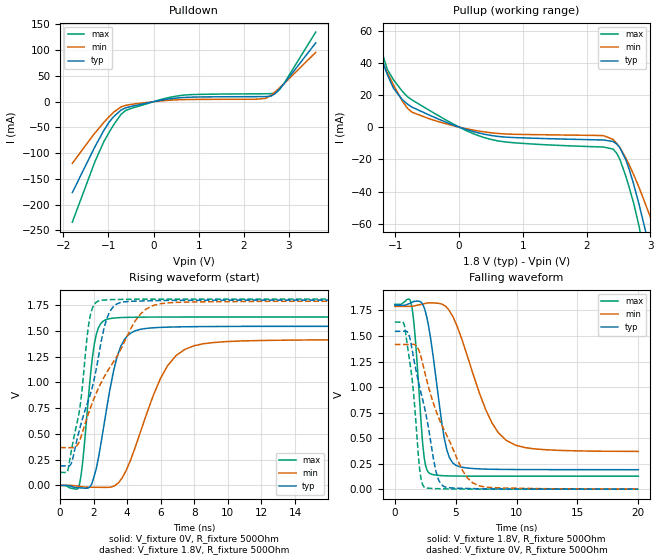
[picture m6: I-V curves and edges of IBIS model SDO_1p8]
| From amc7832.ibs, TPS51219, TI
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|   Model
[Model]   SDO_1p8
Model_type   Output
Polarity   Non-Inverting
Vmeas = 0.9
Vref = 0
Cref = 1pF
Rref = 100000
|   typ   min   max
C_comp   1pF   1pF   1pF
[Voltage Range]   1.8   1.79   1.81
[Temperature Range]   27   125   -40
[Pullup Reference]   1.8   1.79   1.81
[Pulldown Reference]   -0   -0   -0
[Power Clamp Reference]   1.8   1.79   1.81
[GND Clamp Reference]   -0   -0   -0
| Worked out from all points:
|   slope of the pulldown table from 0 to 0.27 V, typ, clamps not added: 62.1 ohm
|   slope of the pullup table from 0 to 0.27 V, typ, clamps not added: 83.4 ohm
|   falling waveform, V_fixture 1.8V, R_fixture 500Ohm: 20-80 % time 1.1ns typ, 2.57ns min, 595ps max; typ from 1.8 V to 0.19 V
|   rising waveform, V_fixture 0V, R_fixture 500Ohm: 20-80 % time 1.05ns typ, 2.02ns min, 575ps max; typ from 0 V to 1.54 V
|   rising waveform, V_fixture 1.8V, R_fixture 500Ohm: 20-80 % time 1.45ns typ, 2.57ns min, 813ps max; typ from 0.191 V to 1.8 V
|   falling waveform, V_fixture 0V, R_fixture 500Ohm: 20-80 % time 1.54ns typ, 2.68ns min, 785ps max; typ from 1.54 V to 0 V
[Pulldown]
|   Voltage   I(typ)   I(min)   I(max)
-1.8V     -176.6mA   -119.8mA   -234.2mA
-1.319V   -91.03mA   -63.11mA   -121.2mA
-1.103V   -56.2mA    -40.42mA   -78.11mA
-882mV    -29.02mA   -20.34mA   -44.72mA
-725.4mV  -16.76mA   -10.41mA   -25.13mA
-617.4mV  -11.91mA   -7.125mA   -16.98mA
608.4mV   7.777mA    3.867mA    12.1mA
2.266V    9.812mA    4.73mA     15.25mA
2.482V    9.901mA    6.398mA    15.37mA
2.704V    16.5mA     19.76mA    17.88mA
2.887V    34.45mA    34.64mA    34.98mA
3.595V    114.2mA    95.9mA     135.2mA
[Pullup]
|   Voltage   I(typ)   I(min)   I(max)
-1.8V     106.2mA    91.41mA    124mA
-1.13V    33.03mA    34.12mA    36.12mA
-1.028V   23.98mA    25.93mA    29.25mA
-741.6mV  12.48mA    9.317mA    16.94mA
79.2mV    -1.059mA   -706.5uA   -1.565mA
532.8mV   -5.359mA   -3.633mA   -7.934mA
2.412V    -8.894mA   -7.573mA   -13.62mA
2.509V    -12.21mA   -12.12mA   -19.05mA
2.617V    -20.57mA   -19.46mA   -30.92mA
2.822V    -48.11mA   -37.54mA   -61.75mA
3.076V    -89.49mA   -63.86mA   -116.8mA
3.595V    -182.3mA   -125mA     -240mA
[Ramp]
R_load = 500
|   typ   min   max
dV/dt_r   0.927288/1.04577e-09   0.849503/2.01972e-09   0.981518/5.74678e-10
dV/dt_f   0.965724/1.10475e-09   0.852348/2.57092e-09   1.00988/5.95424e-10
[Falling Waveform]
V_fixture = 1.8V
V_fixture_min = 1.79V
V_fixture_max = 1.81V
R_fixture = 500Ohm
C_fixture = 0F
|   Time   V(typ)   V(min)   V(max)
0s        1.8V       1.79V      1.81V
1.334ns   1.825V     1.79V      1.823V
1.614ns   1.839V     1.795V     1.565V
2.4ns     1.778V     1.816V     317.3mV
2.878ns   1.519V     1.824V     153.3mV
4.045ns   507.8mV    1.8V       131.3mV
5.031ns   232.3mV    1.619V     128.4mV
7.453ns   196.4mV    782.1mV    127.2mV
9.149ns   193.1mV    478.1mV    126.9mV
20ns      190.5mV    369.4mV    126.9mV
[Rising Waveform]
V_fixture = 0V
V_fixture_min = 0V
V_fixture_max = 0V
R_fixture = 500Ohm
C_fixture = 0F
|   Time   V(typ)   V(min)   V(max)
0s        653.6nV    -4.818uV   -13.58nV
1.125ns   -22.64mV   -8.709mV   -3.057mV
1.334ns   -25.07mV   -13.18mV   212mV
2.041ns   98.51mV    -17.78mV   1.378V
2.639ns   613.2mV    -18.91mV   1.603V
3.389ns   1.247V     14.61mV    1.628V
4.045ns   1.459V     187.9mV    1.632V
5.973ns   1.535V     1.036V     1.635V
7.453ns   1.541V     1.323V     1.636V
20ns      1.545V     1.416V     1.636V
[Rising Waveform]
V_fixture = 1.8V
V_fixture_min = 1.79V
V_fixture_max = 1.81V
R_fixture = 500Ohm
C_fixture = 0F
|   Time   V(typ)   V(min)   V(max)
0s        190.5mV    367.8mV    126.9mV
467.4ps   189.7mV    366.7mV    149.8mV
1.169ns   552mV      438.6mV    746.2mV
1.708ns   839.7mV    708.7mV    1.572V
2.28ns    1.246V     943.2mV    1.791V
2.784ns   1.622V     1.099V     1.802V
3.17ns    1.737V     1.198V     1.805V
4.453ns   1.79V      1.592V     1.809V
5.551ns   1.794V     1.747V     1.809V
20ns      1.8V       1.79V      1.81V
[Falling Waveform]
|Gnd
V_fixture = 0V
V_fixture_min = 0V
V_fixture_max = 0V
R_fixture = 500Ohm
C_fixture = 0F
|   Time   V(typ)   V(min)   V(max)
0s        1.545V     1.417V     1.636V
807.6ps   1.547V     1.416V     1.59V
1.141ns   1.516V     1.417V     1.315V
1.427ns   1.36V      1.419V     1.068V
2.041ns   996.3mV    1.339V     189.1mV
2.4ns     818.1mV    1.173V     22.05mV
3.608ns   86.45mV    698.4mV    4.529mV
5.551ns   7.741mV    184.8mV    1.089mV
6.395ns   5.395mV    62.04mV    640.1uV
20ns      -24.99uV   612.5uV    -33.05nV
